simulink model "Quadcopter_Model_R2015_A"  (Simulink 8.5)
settings: Solver=ode45  SolverMode=SingleTasking  StartTime=0.0  StopTime=runtime  RelTol=1e-3
InitFcn:
  | clear mex
  | delete test_model_sfun.mexw64
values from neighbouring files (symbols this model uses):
  g = 9.81    [modelParameters.m]    (also in analyzeIMU_data.m = 9.8; getMomentOfInertia.m = 9.80665)
  height_controlled_o = dataStruct.RC_Throttle_Constant.data(1)    [modelParameters.m]
  If = 0.3836    [modelParameters.m]    (also in thrustDragConstantCalculations.m = [If0; If1; If2; If3]; Kd_error.m = I_0 * sign(rotor_speed_0) + I_1 * rotor_speed_0 + I_2 * roto)
  Jreq = 4.2012e-05    [modelParameters.m]
  Jxx = 0.0130    (= 0.013)    [modelParameters.m]
  Jyy = 0.0140    (= 0.014)    [modelParameters.m]
  Jzz = 0.0285    [modelParameters.m]
  Kd = 1.4852e-07    [modelParameters.m]    (also in calcDragConstant.m = ((A'*A)^-1)*A'*b; thrustDragConstantCalculations.m = calcDragConstant(data, Pmin, Pmax, Rm, Kv, Kq, If); Kd_error.m = 1.0317e-07)
  Kq = 96.3422    [modelParameters.m]    (also in thrustDragConstantCalculations.m; Kd_error.m)
  Kt = 1.2007e-05    [modelParameters.m]    (also in calcThrustConstant.m = ((A'*A)^(-1))*(A'*T); thrustDragConstantCalculations.m = calcThrustConstant(data))
  Kv = 96.3422    [modelParameters.m]    (also in thrustDragConstantCalculations.m; Kd_error.m)
  m = 1.140    (= 1.14)    [modelParameters.m]
  omega0_o = (sqrt(((height_controlled_o      - Pmin)/(Pmax - Pmin)* Vb - Rm * If) * 4 *      Rm * Kv^2 * Kq * Kd + 1) - 1) / (2 * Rm *       Kv * Kq * Kd)    [modelParameters.m]
  omega1_o = omega0_o    [modelParameters.m]
  omega2_o = omega0_o    [modelParameters.m]
  omega3_o = omega0_o    [modelParameters.m]
  pitch_o = pitch_measured_VRPN(1)    [modelParameters.m]
  pitchrate_o = (pitch_measured_VRPN(1) - pitch_measured_VRPN(2))/(time(1) - time(2))    [modelParameters.m]
  Pmax = 2e5    (= 200000)    [modelParameters.m]    (also in thrustDragConstantCalculations.m; Kd_error.m)
  Pmin = 1e5    (= 100000)    [modelParameters.m]    (also in thrustDragConstantCalculations.m; Kd_error.m)
  rhx = 0.16    [modelParameters.m]
  rhy = 0.16    [modelParameters.m]
  rhz = 0.03    [modelParameters.m]
  Rm = 0.2308    [modelParameters.m]    (also in thrustDragConstantCalculations.m; Kd_error.m)
  roll_o = roll_measured_VRPN(1)    [modelParameters.m]
  rollrate_o = (roll_measured_VRPN(1) - roll_measured_VRPN(2))/(time(1) - time(2))    [modelParameters.m]
  Tc = 0.04    [modelParameters.m]
  Tq = 0.005    [modelParameters.m]
  Vb = 11.4    [modelParameters.m]    (also in calcDragConstant.m = [data.(6); data.(6); data.(6); data.(6)]; Kd_error.m = data.(6))
  x_controlled_o = 0    [modelParameters.m]
  x_o = x_position(1)    [modelParameters.m]
  x_vel_o = (x_position(1) - x_position(2))/(time(1) - time(2))    [modelParameters.m]
  y_controlled_o = 0    [modelParameters.m]
  y_o = y_position(1)    [modelParameters.m]
  y_vel_o = (y_position(1) - y_position(2))/(time(1) - time(2))    [modelParameters.m]
  yaw_controlled_o = 0    [modelParameters.m]
  yaw_o = 0    [modelParameters.m]
  yawrate_o = 0    [modelParameters.m]
  z_o = z_position(1)    [modelParameters.m]
  z_vel_o = (z_position(1) - z_position(2))/(time(1) - time(2))    [modelParameters.m]
undefined symbols (not defined in the file or in its folder): DiscIntNeverNeededParam
libraries: simulink x12, vrlib x2
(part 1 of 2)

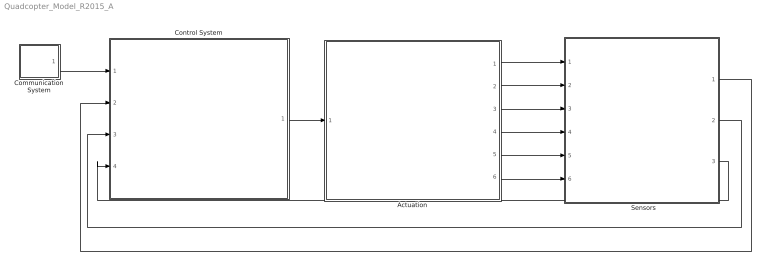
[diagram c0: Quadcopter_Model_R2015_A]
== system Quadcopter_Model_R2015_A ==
  "     Sensors   " : Subsystem
  Actuation : Subsystem
  Communication System : Subsystem
  Control System : Subsystem
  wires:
  Control System/1(P) -> Actuation/1(P)
  Communication System/1(setpoints) -> Control System/1(setpoints)
  Actuation/1(B_omega) -> "     Sensors   "/1(B_Omega)
  Actuation/2(euler_angles) -> "     Sensors   "/2(euler_angles)
  Actuation/3(B_vo) -> "     Sensors   "/3(B_vo)
  Actuation/4(E_ro) -> "     Sensors   "/4(E_ro)
  Actuation/5(B_vo_dot) -> "     Sensors   "/5(B_vo_dot)
  Actuation/6(B_g) -> "     Sensors   "/6(B_g)
  "     Sensors   "/3(current_position) -> Control System/4(current_position)
  "     Sensors   "/2(euler_rates) -> Control System/3(euler_rates)
  "     Sensors   "/1(euler_angles_filtered) -> Control System/2(euler_angles_filtered)

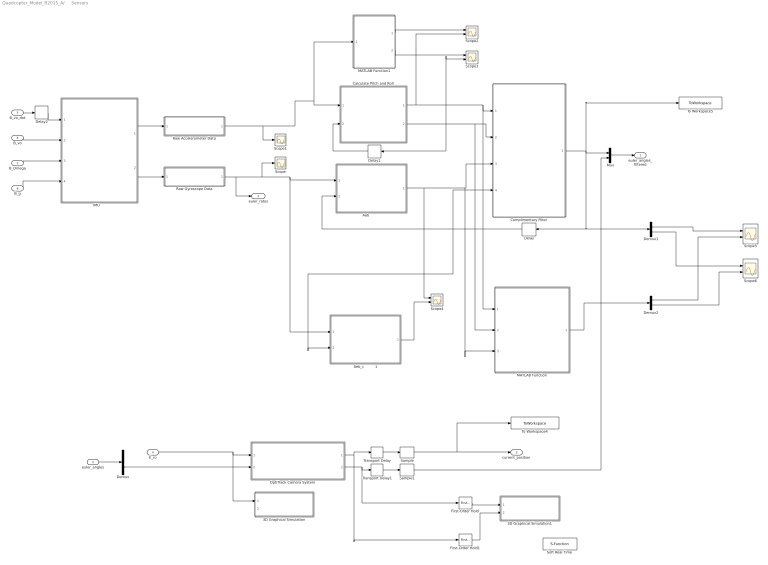
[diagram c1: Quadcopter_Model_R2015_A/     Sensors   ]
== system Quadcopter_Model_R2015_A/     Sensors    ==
  B_Omega : Inport
  euler_angles : Inport  Port=2
  B_vo : Inport  Port=3
  E_ro : Inport  Port=4
  B_vo_dot : Inport  Port=5
  B_g : Inport  Port=6
  3D Graphical Simulation : Subsystem  Commented=on
  3D Graphical Simulation1 : Subsystem  Commented=on
  "Aeb          " : MATLAB Function  TreatAsAtomicUnit=on
  Aeb_c          1 : MATLAB Function  TreatAsAtomicUnit=on
  Calculate Pitch and Roll : MATLAB Function  TreatAsAtomicUnit=on
  Complimentary Filter : MATLAB Function  TreatAsAtomicUnit=on
  Delay : Delay  DelayLength=1  InitialCondition=0
  Delay1 : Delay  DelayLength=1  InitialCondition=0  SampleTime=Tq
  Delay2 : Delay  DelayLength=1  InitialCondition=0  SampleTime=Tq
  Demux : Demux  Outputs=3
  Demux1 : Demux  Outputs=2
  Demux2 : Demux  Outputs=2
  First-Order Hold : simulink/Discrete/First-Order Hold  DisableCoverage=on  Ts=5e-3
  First-Order Hold1 : simulink/Discrete/First-Order Hold  DisableCoverage=on  Ts=5e-3
  "IMU      " : Subsystem
  MATLAB Function : MATLAB Function  TreatAsAtomicUnit=on
  MATLAB Function1 : MATLAB Function  TreatAsAtomicUnit=on
  Mux : Mux  Inputs=2
  "OptiTrack Camera System         " : Subsystem
  Raw Accelerometer Data : Subsystem  Variant=on
  Raw Gyroscope Data : Subsystem  Variant=on
  Sample : ZeroOrderHold  SampleTime=Tc
  Sample1 : ZeroOrderHold  SampleTime=Tc
  Scope : Scope
  Scope1 : Scope
  Scope{2..6} (5 alike) : Scope  NumInputPorts=2
  Soft Real Time : S-Function  Commented=on  FunctionName=sfun_time  Parameters=x  SFunctionDeploymentMode=off  EnableBusSupport=off
  To Workspace4 : ToWorkspace  VariableName=position_model  SaveFormat=Structure With Time  SampleTime=Tc
  To Workspace5 : ToWorkspace  VariableName=angle_IMU_reading  SaveFormat=Structure With Time  SampleTime=Tq
  Transport Delay : TransportDelay  DelayTime=6e-3
  Transport Delay1 : TransportDelay  DelayTime=6e-3
  euler_angles_filtered : Outport
  euler_rates : Outport  Port=2
  current_position : Outport  Port=3
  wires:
  "IMU      "/1(accelerometer) -> Raw Accelerometer Data/1(raw_accel_model)
  "IMU      "/2(gyroscope) -> Raw Gyroscope Data/1(raw_gyro_model)
  B_vo/1 -> "IMU      "/2(B_vo)
  B_Omega/1 -> "IMU      "/3(B_Omega)
  B_g/1 -> "IMU      "/4(B_g)
  Calculate Pitch and Roll/2(accel_roll) -> Scope3/2, Delay1/1, MATLAB Function/2(accel_roll), Complimentary Filter/2(accel_roll)
  Calculate Pitch and Roll/1(accel_pitch) -> Scope2/2, MATLAB Function/1(accel_pitch), Complimentary Filter/1(accel_pitch)
  Delay1/1 -> Calculate Pitch and Roll/2(accel_roll_prev)
  First-Order Hold/1 -> 3D Graphical Simulation1/1("Euler Angles ")
  E_ro/1 -> 3D Graphical Simulation/1(Displacement), "OptiTrack Camera System         "/1(E_ro)
  First-Order Hold1/1 -> 3D Graphical Simulation1/2(Displacement)
  B_vo_dot/1 -> Delay2/1
  Delay2/1 -> "IMU      "/1(B_vo_dot)
  "OptiTrack Camera System         "/1(E_ro_camera) -> Transport Delay/1, First-Order Hold1/1
  "OptiTrack Camera System         "/2(yaw_camera) -> First-Order Hold/1, Transport Delay1/1
  Transport Delay/1 -> Sample/1
  Transport Delay1/1 -> Sample1/1
  Sample/1 -> To Workspace4/1, current_position/1
  Raw Accelerometer Data/1(raw_accel) -> MATLAB Function1/1(accel_reading), Calculate Pitch and Roll/1(accel_reading), Scope1/1
  Raw Gyroscope Data/1(raw_gyro) -> Aeb_c          1/1(gyro_reading), "Aeb          "/1(gyro_reading), Scope/1, euler_rates/1
  Delay/1 -> Complimentary Filter/4(prev_euler_angles), Aeb_c          1/2(euler_angles_filtered), "Aeb          "/2(euler_angles_filtered)
  euler_angles/1 -> Demux/1
  Demux/3 -> "OptiTrack Camera System         "/2(yaw)
  Sample1/1 -> Mux/2
  Mux/1 -> euler_angles_filtered/1
  Complimentary Filter/1(euler_angles_IMU) -> Mux/1, To Workspace5/1, Demux1/1, Delay/1
  "Aeb          "/1(euler_rates_IMU) -> Scope4/1, MATLAB Function/3(euler_rates_gyro), Complimentary Filter/3(euler_rates_gyro)
  Aeb_c          1/1(euler_rates_IMU) -> Scope4/2
  MATLAB Function/1(euler_angles_IMU) -> Demux2/1
  Demux1/1 -> Scope5/1
  Demux2/1 -> Scope5/2
  Demux1/2 -> Scope6/1
  Demux2/2 -> Scope6/2
  MATLAB Function1/1(accel_pitch) -> Scope2/1
  MATLAB Function1/2(accel_roll) -> Scope3/1

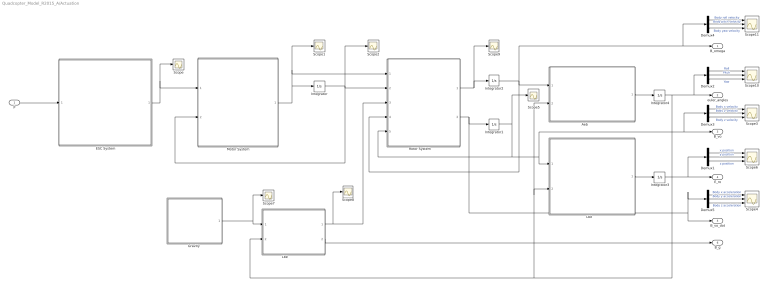
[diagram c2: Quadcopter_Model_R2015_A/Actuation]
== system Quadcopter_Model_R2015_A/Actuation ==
  P : Inport
  "Aeb               " : MATLAB Function  TreatAsAtomicUnit=on
  Demux{1..5} (5 alike) : Demux  Outputs=3
  ESC System : MATLAB Function  TreatAsAtomicUnit=on
  "Gravity  " : MATLAB Function  TreatAsAtomicUnit=on
  Integrator : Integrator  InitialCondition=[omega0_o, omega1_o, omega2_o, omega3_o]
  Integrator1 : Integrator  InitialCondition=[x_vel_o; y_vel_o; z_vel_o]
  Integrator2 : Integrator  InitialCondition=[rollrate_o; pitchrate_o; yawrate_o]
  Integrator3 : Integrator  InitialCondition=[x_o; y_o; z_o]
  Integrator4 : Integrator  InitialCondition=[roll_o; pitch_o; yaw_o]  ContinuousStateAttributes=['phi' 'theta' 'psi']
  "Lbe      " : MATLAB Function  TreatAsAtomicUnit=on
  "Lbe                  " : MATLAB Function  TreatAsAtomicUnit=on
  Motor System : MATLAB Function  TreatAsAtomicUnit=on
  "Rotor System        " : MATLAB Function  TreatAsAtomicUnit=on
  Scope{,1..2,5,7..9} (7 alike) : Scope
  Scope{3..4,6,10..11} (5 alike) : Scope  NumInputPorts=3
  B_omega : Outport
  euler_angles : Outport  Port=2
  B_vo : Outport  Port=3
  E_ro : Outport  Port=4
  B_vo_dot : Outport  Port=5
  B_g : Outport  Port=6
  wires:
  ESC System/1(Vb_eff) -> Scope/1, Motor System/1(Vb_eff)
  Motor System/1(w_dot) -> Integrator/1, "Rotor System        "/1(w_dot), Scope1/1
  "Rotor System        "/1(B_omega_dot) -> Scope9/1, Integrator2/1
  Integrator2/1 -> "Rotor System        "/4(B_omega), B_omega/1, Demux4/1, "Aeb               "/1(B_omega)
  "Aeb               "/1(euler_rates) -> Integrator4/1
  "Lbe      "/1(E_ro) -> Integrator3/1
  Integrator3/1 -> Demux1/1, E_ro/1
  "Lbe                  "/1(B_Fg) -> Scope8/1, "Rotor System        "/3(B_Fg)
  "Lbe                  "/2(B_g) -> B_g/1
  Demux1/2 -> Scope6/2  "y position"
  Demux1/1 -> Scope6/1  "x position"
  Demux1/3 -> Scope6/3  "z position"
  Demux2/2 -> Scope10/2  "Pitch"
  Demux2/1 -> Scope10/1  "Roll"
  Demux2/3 -> Scope10/3  "Yaw"
  Demux4/2 -> Scope11/2  "Body pitch velocity"
  Demux4/1 -> Scope11/1  "Body roll velocity"
  Demux4/3 -> Scope11/3  "Body yaw velocity"
  Demux3/2 -> Scope3/2  "Body y velocity"
  Demux3/1 -> Scope3/1  "Body x velocity"
  Demux3/3 -> Scope3/3  "Body z velocity"
  Demux5/2 -> Scope4/2  "Body y acceleration"
  Demux5/1 -> Scope4/1  "Body x acceleration"
  Demux5/3 -> Scope4/3  "Body z acceleration"
  Integrator1/1 -> Scope5/1, "Rotor System        "/5(B_vo), "Lbe      "/1(B_vo), Demux3/1, B_vo/1
  "Rotor System        "/2(B_vo_dot) -> Demux5/1, B_vo_dot/1, Integrator1/1
  Integrator4/1 -> euler_angles/1, Demux2/1, "Lbe      "/2(euler_angles), "Aeb               "/2(euler_angles), "Lbe                  "/2(euler_angles)
  P/1 -> ESC System/1(P)
  "Gravity  "/1(E_Fg) -> Scope7/1, "Lbe                  "/1(E_Fg)
  Integrator/1 -> Motor System/2(w), "Rotor System        "/2(w), Scope2/1

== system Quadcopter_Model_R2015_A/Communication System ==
  Step : Step  Before=[0; 0; 0; 0]  After=[0; 0; 0; 0]  SampleTime=Tq
  setpoints : Outport
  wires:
  Step/1 -> setpoints/1

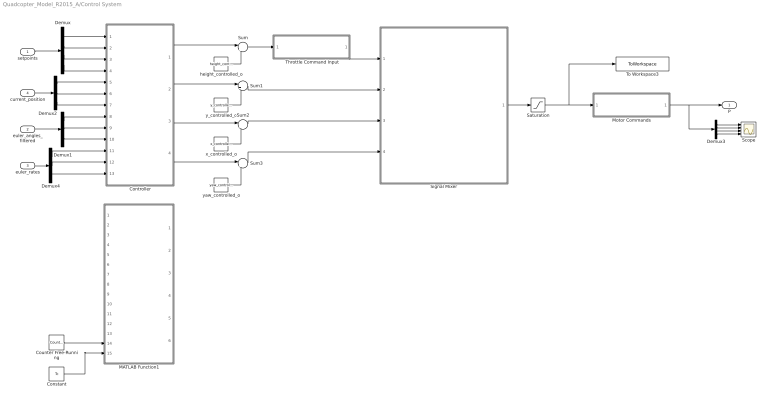
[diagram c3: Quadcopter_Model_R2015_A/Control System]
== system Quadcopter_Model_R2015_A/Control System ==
  setpoints : Inport
  euler_angles_filtered : Inport  Port=2
  euler_rates : Inport  Port=3
  current_position : Inport  Port=4
  Constant : Constant  Value=Tc  SampleTime=Tc
  Controller : Subsystem
  Counter Free-Running : simulink/Sources/Counter Free-Running  NumBits=32  tsamp=Tc
  Demux : Demux
  Demux1 : Demux  Outputs=3
  Demux2 : Demux  Outputs=3
  Demux3 : Demux
  Demux4 : Demux  Outputs=3
  MATLAB Function1 : MATLAB Function  Commented=on  TreatAsAtomicUnit=on  SystemSampleTime=Tq
  Motor Commands : Subsystem  Variant=on
  Saturation : Saturate  UpperLimit=Pmax*ones(4,1)  LowerLimit=Pmin*ones(4,1)
  Scope : Scope  NumInputPorts=4
  Signal Mixer : MATLAB Function  TreatAsAtomicUnit=on
  Sum{,1..3} (4 alike) : Sum  Inputs=|++
  Throttle Command Input : Subsystem  Variant=on
  To Workspace3 : ToWorkspace  VariableName=motorCommands  SaveFormat=Structure With Time  SampleTime=Tq
  height_controlled_o : Constant  Value=height_controlled_o  SampleTime=Tc
  x_controlled_o : Constant  Value=x_controlled_o
  y_controlled_o : Constant  Value=y_controlled_o
  yaw_controlled_o : Constant  Value=yaw_controlled_o
  P : Outport
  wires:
  setpoints/1 -> Demux/1
  euler_angles_filtered/1 -> Demux1/1
  current_position/1 -> Demux2/1
  euler_rates/1 -> Demux4/1
  Demux/1 -> Controller/1(x_setpoint)
  Demux/2 -> Controller/2(y_setpoint)
  Demux/3 -> Controller/3(z_setpoint)
  Demux2/1 -> Controller/5(x_position)
  Demux2/2 -> Controller/6(y_position)
  Demux2/3 -> Controller/7(z_position)
  Controller/2(y_controlled) -> Sum1/1
  Controller/4(yaw_controlled) -> Sum3/1
  y_controlled_o/1 -> Sum1/2
  x_controlled_o/1 -> Sum2/2
  yaw_controlled_o/1 -> Sum3/2
  Signal Mixer/1(P) -> Saturation/1
  Demux1/1 -> Controller/8(roll)
  Demux1/2 -> Controller/9(pitch)
  Demux4/1 -> Controller/11(roll_rate)
  Demux4/2 -> Controller/12(pitch_rate)
  Demux4/3 -> Controller/13(yaw_rate)
  Demux/4 -> Controller/4(yaw_setpoint)
  Demux1/3 -> Controller/10(yaw)
  Controller/3(x_controlled) -> Sum2/1
  Counter Free-Running/1 -> MATLAB Function1/14(vrpn_id)
  Constant/1 -> MATLAB Function1/15(Tc)
  Sum1/1 -> Signal Mixer/2(y_controlled)
  Sum2/1 -> Signal Mixer/3(x_controlled)
  Sum3/1 -> Signal Mixer/4(yaw_controlled)
  Throttle Command Input/1(z_command) -> Signal Mixer/1(height_controlled)
  Controller/1(height_controlled) -> Sum/1
  height_controlled_o/1 -> Sum/2
  Motor Commands/1(z_command) -> Demux3/1, P/1
  Demux3/1 -> Scope/1
  Demux3/2 -> Scope/2
  Demux3/3 -> Scope/3
  Demux3/4 -> Scope/4
  Sum/1 -> Throttle Command Input/1(z_command_model)
  Saturation/1 -> To Workspace3/1, Motor Commands/1(z_command_model)

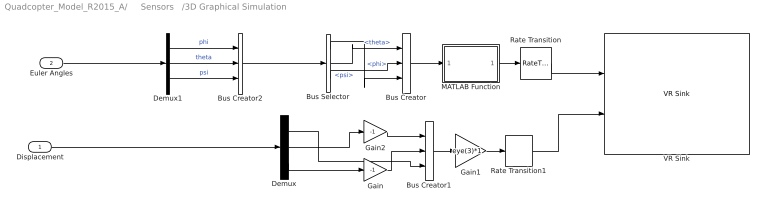
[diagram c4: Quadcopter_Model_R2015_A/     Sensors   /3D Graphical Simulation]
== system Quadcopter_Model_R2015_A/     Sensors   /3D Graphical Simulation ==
  Displacement : Inport
  Euler Angles : Inport  Port=2
  Bus Creator : BusCreator  Inputs=3
  Bus Creator1 : BusCreator  Inputs=3
  Bus Creator2 : BusCreator  Inputs=3
  Bus Selector : BusSelector  OutputSignals=phi,theta,psi
  Demux : Demux  Outputs=3
  Demux1 : Demux  Outputs=3
  Gain : Gain  Gain=-1
  Gain1 : Gain  Gain=eye(3)*1  Multiplication=Matrix(K*u)
  Gain2 : Gain  Gain=-1
  MATLAB Function : MATLAB Function  TreatAsAtomicUnit=on
  Rate Transition : RateTransition  OutPortSampleTime=0.06
  Rate Transition1 : RateTransition  OutPortSampleTime=0.06
  VR Sink : vrlib/VR Sink  InstantiateOnLoad=on  SampleTime=-1  ViewEnable=on  RemoteChange=off  RemoteView=off  FieldsWritten=Helicopter.rotation.4.1.1.double#Helicopter.translation.3.1.1.double  WorldFileName=quadrotor_world_ucart.wrl  AutoView=on  VideoDimensions=[]  AllowVariableSize=off
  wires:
  Displacement/1 -> Demux/1
  Bus Creator2/1 -> Bus Selector/1
  Demux/1 -> Bus Creator1/3
  Gain/1 -> Bus Creator1/2
  Gain2/1 -> Bus Creator1/1
  Rate Transition1/1 -> VR Sink/2
  Rate Transition/1 -> VR Sink/1
  Demux/3 -> Gain/1
  Demux/2 -> Gain2/1
  Bus Creator1/1 -> Gain1/1
  Bus Selector/1 -> Bus Creator/3  "<phi>"
  Bus Selector/3 -> Bus Creator/2  "<psi>"
  Bus Selector/2 -> Bus Creator/1  "<theta>"
  Gain1/1 -> Rate Transition1/1
  Demux1/3 -> Bus Creator2/3  "psi"
  Demux1/2 -> Bus Creator2/2  "theta"
  Demux1/1 -> Bus Creator2/1  "phi"
  Euler Angles/1 -> Demux1/1
  Bus Creator/1 -> MATLAB Function/1(u)
  MATLAB Function/1(y) -> Rate Transition/1

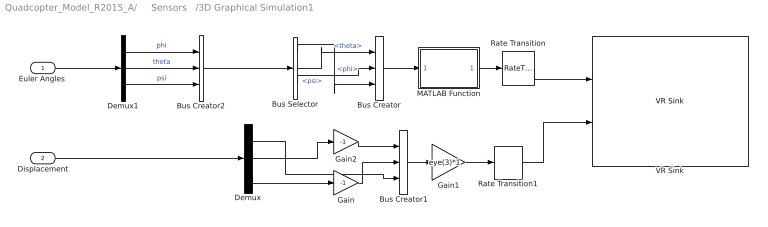
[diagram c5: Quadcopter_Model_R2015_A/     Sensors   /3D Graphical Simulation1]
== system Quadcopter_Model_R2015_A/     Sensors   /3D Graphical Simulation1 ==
  "Euler Angles " : Inport
  Displacement : Inport  Port=2
  Bus Creator : BusCreator  Inputs=3
  Bus Creator1 : BusCreator  Inputs=3
  Bus Creator2 : BusCreator  Inputs=3
  Bus Selector : BusSelector  OutputSignals=phi,theta,psi
  Demux : Demux  Outputs=3
  Demux1 : Demux  Outputs=3
  Gain : Gain  Gain=-1
  Gain1 : Gain  Gain=eye(3)*1  Multiplication=Matrix(K*u)
  Gain2 : Gain  Gain=-1
  MATLAB Function : MATLAB Function  TreatAsAtomicUnit=on
  Rate Transition : RateTransition  OutPortSampleTime=0.06
  Rate Transition1 : RateTransition  OutPortSampleTime=0.06
  VR Sink : vrlib/VR Sink  InstantiateOnLoad=on  SampleTime=-1  ViewEnable=on  RemoteChange=off  RemoteView=off  FieldsWritten=Helicopter.rotation.4.1.1.double#Helicopter.translation.3.1.1.double  WorldFileName=quadrotor_world_ucart.wrl  AutoView=on  VideoDimensions=[]  AllowVariableSize=off
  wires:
  Bus Creator2/1 -> Bus Selector/1
  Demux/1 -> Bus Creator1/3
  Gain/1 -> Bus Creator1/2
  Gain2/1 -> Bus Creator1/1
  Rate Transition1/1 -> VR Sink/2
  Rate Transition/1 -> VR Sink/1
  Demux/3 -> Gain/1
  Demux/2 -> Gain2/1
  Bus Creator1/1 -> Gain1/1
  Bus Selector/1 -> Bus Creator/3  "<phi>"
  Bus Selector/3 -> Bus Creator/2  "<psi>"
  Bus Selector/2 -> Bus Creator/1  "<theta>"
  Gain1/1 -> Rate Transition1/1
  Demux1/3 -> Bus Creator2/3  "psi"
  Demux1/2 -> Bus Creator2/2  "theta"
  Demux1/1 -> Bus Creator2/1  "phi"
  Bus Creator/1 -> MATLAB Function/1(u)
  MATLAB Function/1(y) -> Rate Transition/1
  Displacement/1 -> Demux/1
  "Euler Angles "/1 -> Demux1/1

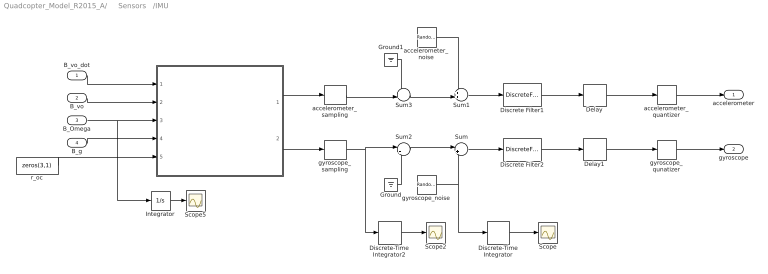
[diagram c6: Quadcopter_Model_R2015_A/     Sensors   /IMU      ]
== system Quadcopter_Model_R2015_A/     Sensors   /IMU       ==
  B_vo_dot : Inport
  B_vo : Inport  Port=2
  B_Omega : Inport  Port=3
  B_g : Inport  Port=4
  "       " : MATLAB Function  TreatAsAtomicUnit=on
  Delay : Delay  Commented=through  DelayLength=4  InitialCondition=0  SampleTime=Tq
  Delay1 : Delay  Commented=through  DelayLength=4  InitialCondition=0  SampleTime=Tq
  Discrete Filter1 : DiscreteFilter  Numerator=[0 0.1454]  Denominator=[1 -0.8546]  InitialStates=[0, 0, -1]  SampleTime=Tq
  Discrete Filter2 : DiscreteFilter  Numerator=[0 0.1454]  Denominator=[1 -0.8546]  SampleTime=Tq
  Discrete-Time Integrator : DiscreteIntegrator  InitialConditionSetting=State (most efficient)  SampleTime=-1  ICPrevOutput=DiscIntNeverNeededParam  ICPrevScaledInput=DiscIntNeverNeededParam
  Discrete-Time Integrator2 : DiscreteIntegrator  InitialConditionSetting=State (most efficient)  SampleTime=-1  ICPrevOutput=DiscIntNeverNeededParam  ICPrevScaledInput=DiscIntNeverNeededParam
  Ground : Ground
  Ground1 : Ground
  Integrator : Integrator
  Scope : Scope
  Scope2 : Scope
  Scope5 : Scope
  Sum : Sum  Inputs=|++
  Sum1 : Sum  Inputs=++|
  Sum2 : Sum  Inputs=|++
  Sum3 : Sum  Inputs=++|
  accelerometer_noise : RandomNumber  Mean=zeros(3,1)  Variance=[ 3e-7 ; 3.3e-7 ; 7.2e-7 ]  Seed=[0,1,2]  SampleTime=Tq
  accelerometer_quantizer : Quantizer  QuantizationInterval=2.4400e-04
  accelerometer_sampling : ZeroOrderHold  SampleTime=Tq
  gyroscope_noise : RandomNumber  Mean=zeros(3,1)  Variance=[ 2.2e-8 ; 1.1e-7 ; 2.4e-8 ]  Seed=[0,1,2]  SampleTime=Tq
  gyroscope_qunatizer : Quantizer  QuantizationInterval=1.1e-3
  gyroscope_sampling : ZeroOrderHold  SampleTime=Tq
  r_oc : Constant  Value=zeros(3,1)
  accelerometer : Outport
  gyroscope : Outport  Port=2
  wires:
  accelerometer_noise/1 -> Sum1/1
  Sum2/1 -> Sum/1
  Sum3/1 -> Sum1/2
  gyroscope_noise/1 -> Sum/2, Discrete-Time Integrator/1
  gyroscope_sampling/1 -> Sum2/1, Discrete-Time Integrator2/1
  accelerometer_sampling/1 -> Sum3/2
  Ground/1 -> Sum2/2
  Ground1/1 -> Sum3/1
  B_vo_dot/1 -> "       "/1(B_vo_dot)
  B_vo/1 -> "       "/2(B_vo)
  B_Omega/1 -> Integrator/1, "       "/3(B_Omega)
  B_g/1 -> "       "/4(B_g)
  r_oc/1 -> "       "/5(r_oc)
  "       "/2(gyroReading) -> gyroscope_sampling/1
  "       "/1(accelReading) -> accelerometer_sampling/1
  Discrete-Time Integrator/1 -> Scope/1
  Discrete-Time Integrator2/1 -> Scope2/1
  Integrator/1 -> Scope5/1
  Sum1/1 -> Discrete Filter1/1
  Sum/1 -> Discrete Filter2/1
  accelerometer_quantizer/1 -> accelerometer/1
  gyroscope_qunatizer/1 -> gyroscope/1
  Discrete Filter1/1 -> Delay/1
  Discrete Filter2/1 -> Delay1/1
  Delay/1 -> accelerometer_quantizer/1
  Delay1/1 -> gyroscope_qunatizer/1

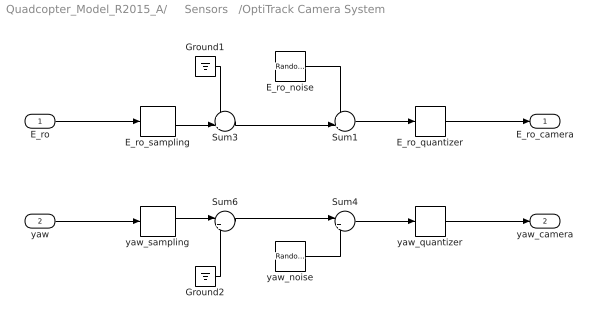
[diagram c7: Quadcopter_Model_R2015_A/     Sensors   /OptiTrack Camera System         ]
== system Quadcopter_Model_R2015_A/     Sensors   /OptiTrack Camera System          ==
  E_ro : Inport
  yaw : Inport  Port=2
  E_ro_noise : RandomNumber  Mean=zeros(3,1)  Variance=[ 7.9664e-10 ; 1.1928e-10 ; 5.0636e-10 ]  Seed=[0,1,2]  SampleTime=Tc
  E_ro_quantizer : Quantizer  QuantizationInterval=2.4400e-04
  E_ro_sampling : ZeroOrderHold  SampleTime=Tc
  Ground1 : Ground
  Ground2 : Ground
  Sum1 : Sum  Inputs=++|
  Sum3 : Sum  Inputs=++|
  Sum4 : Sum  Inputs=|++
  Sum6 : Sum  Inputs=|++
  yaw_noise : RandomNumber  Variance=1.0783e-9  SampleTime=Tc
  yaw_quantizer : Quantizer  QuantizationInterval=1.1e-3
  yaw_sampling : ZeroOrderHold  SampleTime=Tc
  E_ro_camera : Outport
  yaw_camera : Outport  Port=2
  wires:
  E_ro_noise/1 -> Sum1/1
  Sum3/1 -> Sum1/2
  Sum1/1 -> E_ro_quantizer/1
  E_ro_sampling/1 -> Sum3/2
  Ground1/1 -> Sum3/1
  Sum4/1 -> yaw_quantizer/1
  Sum6/1 -> Sum4/1
  yaw_noise/1 -> Sum4/2
  yaw_sampling/1 -> Sum6/1
  Ground2/1 -> Sum6/2
  yaw/1 -> yaw_sampling/1
  E_ro/1 -> E_ro_sampling/1
  E_ro_quantizer/1 -> E_ro_camera/1
  yaw_quantizer/1 -> yaw_camera/1

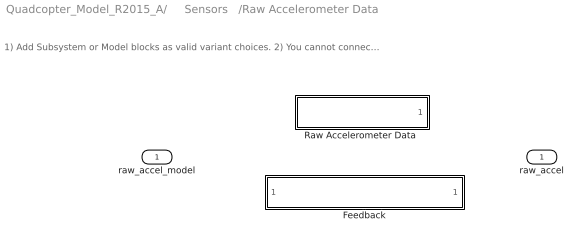
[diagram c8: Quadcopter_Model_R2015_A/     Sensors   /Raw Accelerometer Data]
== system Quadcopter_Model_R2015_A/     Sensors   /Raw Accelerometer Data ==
  note: 1) Add Subsystem or Model blocks as valid variant choices. 2) You cannot connect blocks at this level. At simulation, connectivity is automatically determined, based on the active variant and port name matching.
  raw_accel_model : Inport
  Feedback : Subsystem  VariantControl=logAnalysisToggle==0
  "Raw Accelerometer Data " : Subsystem  VariantControl=logAnalysisToggle==1
  raw_accel : Outport

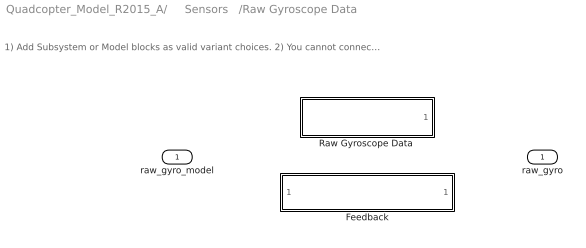
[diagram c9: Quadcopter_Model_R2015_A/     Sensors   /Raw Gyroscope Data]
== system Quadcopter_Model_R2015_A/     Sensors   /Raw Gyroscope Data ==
  note: 1) Add Subsystem or Model blocks as valid variant choices. 2) You cannot connect blocks at this level. At simulation, connectivity is automatically determined, based on the active variant and port name matching.
  raw_gyro_model : Inport
  Feedback : Subsystem  VariantControl=logAnalysisToggle==0
  "Raw Gyroscope Data " : Subsystem  VariantControl=logAnalysisToggle==1
  raw_gyro : Outport

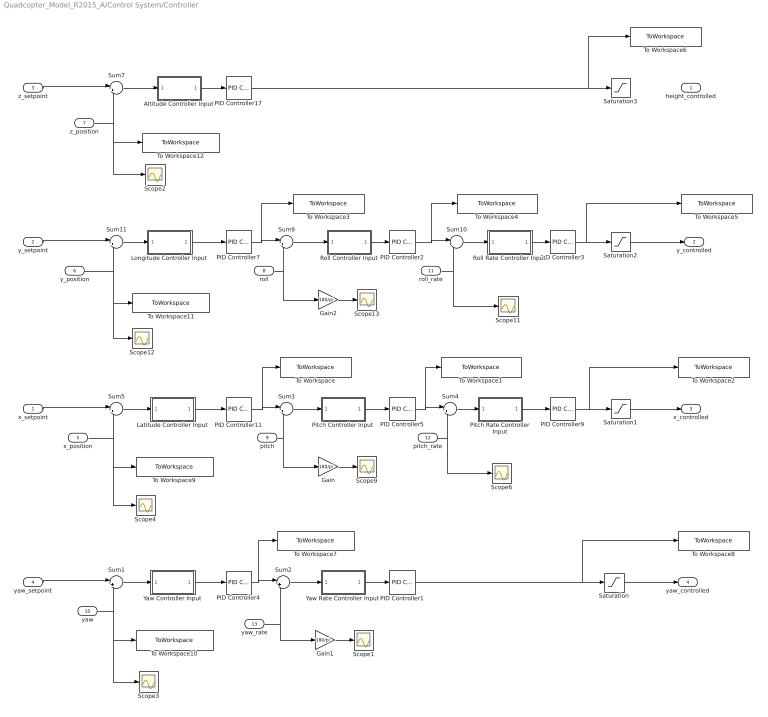
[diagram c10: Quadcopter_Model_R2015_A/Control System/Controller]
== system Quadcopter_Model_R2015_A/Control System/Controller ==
  x_setpoint : Inport
  y_setpoint : Inport  Port=2
  z_setpoint : Inport  Port=3
  yaw_setpoint : Inport  Port=4
  x_position : Inport  Port=5
  y_position : Inport  Port=6
  z_position : Inport  Port=7
  roll : Inport  Port=8
  pitch : Inport  Port=9
  yaw : Inport  Port=10
  roll_rate : Inport  Port=11
  pitch_rate : Inport  Port=12
  yaw_rate : Inport  Port=13
  Altitude Controller Input : Subsystem  Variant=on
  Gain : Gain  Gain=180/pi
  Gain1 : Gain  Gain=180/pi
  Gain2 : Gain  Gain=180/pi
  Latitude Controller Input : Subsystem  Variant=on
  Longitude Controller Input : Subsystem  Variant=on
  PID Controller1 : simulink/Continuous/PID Controller  Controller=P  TimeDomain=Discrete-time  SampleTime=Tq  IntegratorMethod=Forward Euler  FilterMethod=Forward Euler  Form=Parallel  UseFilter=on  ControllerParametersSource=internal  P=29700  I=-77.7  D=2.32  N=1/0.0818  InitialConditionSource=internal  InitialConditionForIntegrator=0  InitialConditionForFilter=0  ExternalReset=none  ZeroCross=off  LimitOutput=off  UpperSaturationLimit=inf  LowerSaturationLimit=-inf  LinearizeAsGain=on  AntiWindupMode=none  Kb=1  TrackingMode=off  Kt=1  PParamMin=[]  PParamMax=[]  IParamMin=[]  IParamMax=[]  DParamMin=[]  DParamMax=[]  NParamMin=[]  NParamMax=[]  KbParamMin=[]  KbParamMax=[]  KtParamMin=[]  KtParamMax=[]  POutMin=[]  POutMax=[]  IOutMin=[]  IOutMax=[]  DOutMin=[]  DOutMax=[]  NOutMin=[]  NOutMax=[]  KbOutMin=[]  KbOutMax=[]  KtOutMin=[]  KtOutMax=[]  IntegratorOutMin=[]  IntegratorOutMax=[]  FilterOutMin=[]  FilterOutMax=[]  SumOutMin=[]  SumOutMax=[]  SumI1OutMin=[]  SumI1OutMax=[]  SumI2OutMin=[]  SumI2OutMax=[]  SumI3OutMin=[]  SumI3OutMax=[]  SumDOutMin=[]  SumDOutMax=[]  SaturationOutMin=[]  SaturationOutMax=[]  IntegratorContinuousStateAttributes=''  IntegratorStateMustResolveToSignalObject=off  IntegratorRTWStateStorageClass=Auto  FilterContinuousStateAttributes=''  FilterStateMustResolveToSignalObject=off  FilterRTWStateStorageClass=Auto  DifferentiatorICPrevScaledInput=0  DifferentiatorOutMin=[]  DifferentiatorOutMax=[]
  PID Controller11 : simulink/Continuous/PID Controller  Controller=PID  TimeDomain=Discrete-time  SampleTime=Tc  IntegratorMethod=Forward Euler  FilterMethod=Forward Euler  Form=Parallel  UseFilter=on  ControllerParametersSource=internal  P=-0.015  I=0  D=-0.25  N=3  InitialConditionSource=internal  InitialConditionForIntegrator=0  InitialConditionForFilter=0  ExternalReset=none  LimitOutput=off  UpperSaturationLimit=inf  LowerSaturationLimit=-inf  LinearizeAsGain=on  AntiWindupMode=none  Kb=1  TrackingMode=off  Kt=1  PParamMin=[]  PParamMax=[]  IParamMin=[]  IParamMax=[]  DParamMin=[]  DParamMax=[]  NParamMin=[]  NParamMax=[]  KbParamMin=[]  KbParamMax=[]  KtParamMin=[]  KtParamMax=[]  POutMin=[]  POutMax=[]  IOutMin=[]  IOutMax=[]  DOutMin=[]  DOutMax=[]  NOutMin=[]  NOutMax=[]  KbOutMin=[]  KbOutMax=[]  KtOutMin=[]  KtOutMax=[]  IntegratorOutMin=[]  IntegratorOutMax=[]  FilterOutMin=[]  FilterOutMax=[]  SumOutMin=[]  SumOutMax=[]  SumI1OutMin=[]  SumI1OutMax=[]  SumI2OutMin=[]  SumI2OutMax=[]  SumI3OutMin=[]  SumI3OutMax=[]  SumDOutMin=[]  SumDOutMax=[]  SaturationOutMin=[]  SaturationOutMax=[]  IntegratorContinuousStateAttributes=''  IntegratorStateMustResolveToSignalObject=off  IntegratorRTWStateStorageClass=Auto  FilterContinuousStateAttributes=''  FilterStateMustResolveToSignalObject=off  FilterRTWStateStorageClass=Auto  DifferentiatorICPrevScaledInput=0  DifferentiatorOutMin=[]  DifferentiatorOutMax=[]
  PID Controller17 : simulink/Continuous/PID Controller  Controller=PID  TimeDomain=Discrete-time  SampleTime=Tc  IntegratorMethod=Forward Euler  FilterMethod=Forward Euler  Form=Parallel  UseFilter=off  ControllerParametersSource=internal  P=9804  I=817  D=7353  N=5.79502261645411  InitialConditionSource=internal  InitialConditionForIntegrator=0  InitialConditionForFilter=0  ExternalReset=none  LimitOutput=off  UpperSaturationLimit=inf  LowerSaturationLimit=-inf  LinearizeAsGain=on  AntiWindupMode=none  Kb=1  TrackingMode=off  Kt=1  PParamMin=[]  PParamMax=[]  IParamMin=[]  IParamMax=[]  DParamMin=[]  DParamMax=[]  NParamMin=[]  NParamMax=[]  KbParamMin=[]  KbParamMax=[]  KtParamMin=[]  KtParamMax=[]  POutMin=[]  POutMax=[]  IOutMin=[]  IOutMax=[]  DOutMin=[]  DOutMax=[]  NOutMin=[]  NOutMax=[]  KbOutMin=[]  KbOutMax=[]  KtOutMin=[]  KtOutMax=[]  IntegratorOutMin=[]  IntegratorOutMax=[]  FilterOutMin=[]  FilterOutMax=[]  SumOutMin=[]  SumOutMax=[]  SumI1OutMin=[]  SumI1OutMax=[]  SumI2OutMin=[]  SumI2OutMax=[]  SumI3OutMin=[]  SumI3OutMax=[]  SumDOutMin=[]  SumDOutMax=[]  SaturationOutMin=[]  SaturationOutMax=[]  IntegratorContinuousStateAttributes=''  IntegratorStateMustResolveToSignalObject=off  IntegratorRTWStateStorageClass=Auto  FilterContinuousStateAttributes=''  FilterStateMustResolveToSignalObject=off  FilterRTWStateStorageClass=Auto  DifferentiatorICPrevScaledInput=0  DifferentiatorOutMin=[]  DifferentiatorOutMax=[]
  PID Controller2 : simulink/Continuous/PID Controller  Controller=PD  TimeDomain=Discrete-time  SampleTime=Tq  IntegratorMethod=Forward Euler  FilterMethod=Forward Euler  Form=Parallel  UseFilter=off  ControllerParametersSource=internal  P=15  I=35.1207902652377  D=0.2  N=40.0107970227961  InitialConditionSource=internal  InitialConditionForIntegrator=0  InitialConditionForFilter=0  ExternalReset=none  LimitOutput=off  UpperSaturationLimit=inf  LowerSaturationLimit=-inf  LinearizeAsGain=on  AntiWindupMode=none  Kb=1  TrackingMode=off  Kt=1  PParamMin=[]  PParamMax=[]  IParamMin=[]  IParamMax=[]  DParamMin=[]  DParamMax=[]  NParamMin=[]  NParamMax=[]  KbParamMin=[]  KbParamMax=[]  KtParamMin=[]  KtParamMax=[]  POutMin=[]  POutMax=[]  IOutMin=[]  IOutMax=[]  DOutMin=[]  DOutMax=[]  NOutMin=[]  NOutMax=[]  KbOutMin=[]  KbOutMax=[]  KtOutMin=[]  KtOutMax=[]  IntegratorOutMin=[]  IntegratorOutMax=[]  FilterOutMin=[]  FilterOutMax=[]  SumOutMin=[]  SumOutMax=[]  SumI1OutMin=[]  SumI1OutMax=[]  SumI2OutMin=[]  SumI2OutMax=[]  SumI3OutMin=[]  SumI3OutMax=[]  SumDOutMin=[]  SumDOutMax=[]  SaturationOutMin=[]  SaturationOutMax=[]  IntegratorContinuousStateAttributes=''  IntegratorStateMustResolveToSignalObject=off  IntegratorRTWStateStorageClass=Auto  FilterContinuousStateAttributes=''  FilterStateMustResolveToSignalObject=off  FilterRTWStateStorageClass=Auto  DifferentiatorICPrevScaledInput=0  DifferentiatorOutMin=[]  DifferentiatorOutMax=[]
  PID Controller3 : simulink/Continuous/PID Controller  Controller=PD  TimeDomain=Discrete-time  SampleTime=Tq  IntegratorMethod=Forward Euler  FilterMethod=Forward Euler  Form=Parallel  UseFilter=off  ControllerParametersSource=internal  P=4600  I=1575.82088970639  D=550  N=244.660686071579  InitialConditionSource=internal  InitialConditionForIntegrator=0  InitialConditionForFilter=0  ExternalReset=none  LimitOutput=off  UpperSaturationLimit=inf  LowerSaturationLimit=-inf  LinearizeAsGain=on  AntiWindupMode=none  Kb=1  TrackingMode=off  Kt=1  PParamMin=[]  PParamMax=[]  IParamMin=[]  IParamMax=[]  DParamMin=[]  DParamMax=[]  NParamMin=[]  NParamMax=[]  KbParamMin=[]  KbParamMax=[]  KtParamMin=[]  KtParamMax=[]  POutMin=[]  POutMax=[]  IOutMin=[]  IOutMax=[]  DOutMin=[]  DOutMax=[]  NOutMin=[]  NOutMax=[]  KbOutMin=[]  KbOutMax=[]  KtOutMin=[]  KtOutMax=[]  IntegratorOutMin=[]  IntegratorOutMax=[]  FilterOutMin=[]  FilterOutMax=[]  SumOutMin=[]  SumOutMax=[]  SumI1OutMin=[]  SumI1OutMax=[]  SumI2OutMin=[]  SumI2OutMax=[]  SumI3OutMin=[]  SumI3OutMax=[]  SumDOutMin=[]  SumDOutMax=[]  SaturationOutMin=[]  SaturationOutMax=[]  IntegratorContinuousStateAttributes=''  IntegratorStateMustResolveToSignalObject=off  IntegratorRTWStateStorageClass=Auto  FilterContinuousStateAttributes=''  FilterStateMustResolveToSignalObject=off  FilterRTWStateStorageClass=Auto  DifferentiatorICPrevScaledInput=0  DifferentiatorOutMin=[]  DifferentiatorOutMax=[]
  PID Controller4 : simulink/Continuous/PID Controller  Controller=PD  TimeDomain=Discrete-time  SampleTime=Tc  IntegratorMethod=Forward Euler  FilterMethod=Forward Euler  Form=Parallel  UseFilter=off  ControllerParametersSource=internal  P=2.6  I=2.36803176515497  D=0  N=3.83298618768959  InitialConditionSource=internal  InitialConditionForIntegrator=0  InitialConditionForFilter=0  ExternalReset=none  LimitOutput=off  UpperSaturationLimit=inf  LowerSaturationLimit=-inf  LinearizeAsGain=on  AntiWindupMode=none  Kb=1  TrackingMode=off  Kt=1  PParamMin=[]  PParamMax=[]  IParamMin=[]  IParamMax=[]  DParamMin=[]  DParamMax=[]  NParamMin=[]  NParamMax=[]  KbParamMin=[]  KbParamMax=[]  KtParamMin=[]  KtParamMax=[]  POutMin=[]  POutMax=[]  IOutMin=[]  IOutMax=[]  DOutMin=[]  DOutMax=[]  NOutMin=[]  NOutMax=[]  KbOutMin=[]  KbOutMax=[]  KtOutMin=[]  KtOutMax=[]  IntegratorOutMin=[]  IntegratorOutMax=[]  FilterOutMin=[]  FilterOutMax=[]  SumOutMin=[]  SumOutMax=[]  SumI1OutMin=[]  SumI1OutMax=[]  SumI2OutMin=[]  SumI2OutMax=[]  SumI3OutMin=[]  SumI3OutMax=[]  SumDOutMin=[]  SumDOutMax=[]  SaturationOutMin=[]  SaturationOutMax=[]  IntegratorContinuousStateAttributes=''  IntegratorStateMustResolveToSignalObject=off  IntegratorRTWStateStorageClass=Auto  FilterContinuousStateAttributes=''  FilterStateMustResolveToSignalObject=off  FilterRTWStateStorageClass=Auto  DifferentiatorICPrevScaledInput=0  DifferentiatorOutMin=[]  DifferentiatorOutMax=[]
  PID Controller5 : simulink/Continuous/PID Controller  Controller=PD  TimeDomain=Discrete-time  SampleTime=Tq  IntegratorMethod=Forward Euler  FilterMethod=Forward Euler  Form=Parallel  UseFilter=off  ControllerParametersSource=internal  P=15  I=35.1207902652377  D=0.2  N=40.0107970227961  InitialConditionSource=internal  InitialConditionForIntegrator=0  InitialConditionForFilter=0  ExternalReset=none  LimitOutput=off  UpperSaturationLimit=inf  LowerSaturationLimit=-inf  LinearizeAsGain=on  AntiWindupMode=none  Kb=1  TrackingMode=off  Kt=1  PParamMin=[]  PParamMax=[]  IParamMin=[]  IParamMax=[]  DParamMin=[]  DParamMax=[]  NParamMin=[]  NParamMax=[]  KbParamMin=[]  KbParamMax=[]  KtParamMin=[]  KtParamMax=[]  POutMin=[]  POutMax=[]  IOutMin=[]  IOutMax=[]  DOutMin=[]  DOutMax=[]  NOutMin=[]  NOutMax=[]  KbOutMin=[]  KbOutMax=[]  KtOutMin=[]  KtOutMax=[]  IntegratorOutMin=[]  IntegratorOutMax=[]  FilterOutMin=[]  FilterOutMax=[]  SumOutMin=[]  SumOutMax=[]  SumI1OutMin=[]  SumI1OutMax=[]  SumI2OutMin=[]  SumI2OutMax=[]  SumI3OutMin=[]  SumI3OutMax=[]  SumDOutMin=[]  SumDOutMax=[]  SaturationOutMin=[]  SaturationOutMax=[]  IntegratorContinuousStateAttributes=''  IntegratorStateMustResolveToSignalObject=off  IntegratorRTWStateStorageClass=Auto  FilterContinuousStateAttributes=''  FilterStateMustResolveToSignalObject=off  FilterRTWStateStorageClass=Auto  DifferentiatorICPrevScaledInput=0  DifferentiatorOutMin=[]  DifferentiatorOutMax=[]
  PID Controller7 : simulink/Continuous/PID Controller  Controller=PID  TimeDomain=Discrete-time  SampleTime=Tc  IntegratorMethod=Forward Euler  FilterMethod=Forward Euler  Form=Parallel  UseFilter=on  ControllerParametersSource=internal  P=0.015  I=0  D=0.25  N=3  InitialConditionSource=internal  InitialConditionForIntegrator=0  InitialConditionForFilter=0  ExternalReset=none  LimitOutput=off  UpperSaturationLimit=inf  LowerSaturationLimit=-inf  LinearizeAsGain=on  AntiWindupMode=none  Kb=1  TrackingMode=off  Kt=1  PParamMin=[]  PParamMax=[]  IParamMin=[]  IParamMax=[]  DParamMin=[]  DParamMax=[]  NParamMin=[]  NParamMax=[]  KbParamMin=[]  KbParamMax=[]  KtParamMin=[]  KtParamMax=[]  POutMin=[]  POutMax=[]  IOutMin=[]  IOutMax=[]  DOutMin=[]  DOutMax=[]  NOutMin=[]  NOutMax=[]  KbOutMin=[]  KbOutMax=[]  KtOutMin=[]  KtOutMax=[]  IntegratorOutMin=[]  IntegratorOutMax=[]  FilterOutMin=[]  FilterOutMax=[]  SumOutMin=[]  SumOutMax=[]  SumI1OutMin=[]  SumI1OutMax=[]  SumI2OutMin=[]  SumI2OutMax=[]  SumI3OutMin=[]  SumI3OutMax=[]  SumDOutMin=[]  SumDOutMax=[]  SaturationOutMin=[]  SaturationOutMax=[]  IntegratorContinuousStateAttributes=''  IntegratorStateMustResolveToSignalObject=off  IntegratorRTWStateStorageClass=Auto  FilterContinuousStateAttributes=''  FilterStateMustResolveToSignalObject=off  FilterRTWStateStorageClass=Auto  DifferentiatorICPrevScaledInput=0  DifferentiatorOutMin=[]  DifferentiatorOutMax=[]
  PID Controller9 : simulink/Continuous/PID Controller  Controller=PD  TimeDomain=Discrete-time  SampleTime=Tq  IntegratorMethod=Forward Euler  FilterMethod=Forward Euler  Form=Parallel  UseFilter=off  ControllerParametersSource=internal  P=4600  I=1575.82088970639  D=550  N=244.660686071579  InitialConditionSource=internal  InitialConditionForIntegrator=0  InitialConditionForFilter=0  ExternalReset=none  LimitOutput=off  UpperSaturationLimit=inf  LowerSaturationLimit=-inf  LinearizeAsGain=on  AntiWindupMode=none  Kb=1  TrackingMode=off  Kt=1  PParamMin=[]  PParamMax=[]  IParamMin=[]  IParamMax=[]  DParamMin=[]  DParamMax=[]  NParamMin=[]  NParamMax=[]  KbParamMin=[]  KbParamMax=[]  KtParamMin=[]  KtParamMax=[]  POutMin=[]  POutMax=[]  IOutMin=[]  IOutMax=[]  DOutMin=[]  DOutMax=[]  NOutMin=[]  NOutMax=[]  KbOutMin=[]  KbOutMax=[]  KtOutMin=[]  KtOutMax=[]  IntegratorOutMin=[]  IntegratorOutMax=[]  FilterOutMin=[]  FilterOutMax=[]  SumOutMin=[]  SumOutMax=[]  SumI1OutMin=[]  SumI1OutMax=[]  SumI2OutMin=[]  SumI2OutMax=[]  SumI3OutMin=[]  SumI3OutMax=[]  SumDOutMin=[]  SumDOutMax=[]  SaturationOutMin=[]  SaturationOutMax=[]  IntegratorContinuousStateAttributes=''  IntegratorStateMustResolveToSignalObject=off  IntegratorRTWStateStorageClass=Auto  FilterContinuousStateAttributes=''  FilterStateMustResolveToSignalObject=off  FilterRTWStateStorageClass=Auto  DifferentiatorICPrevScaledInput=0  DifferentiatorOutMin=[]  DifferentiatorOutMax=[]
  Pitch Controller Input : Subsystem  Variant=on
  Pitch Rate Controller Input : Subsystem  Variant=on
  Roll Controller Input : Subsystem  Variant=on
  Roll Rate Controller Input : Subsystem  Variant=on
  Saturation{,1..3} (4 alike) : Saturate  UpperLimit=20000  LowerLimit=-20000
  Scope{1..4,6,9,11..13} (9 alike) : Scope
  Sum{1..5,7,9..11} (9 alike) : Sum  Inputs=|+-
  To Workspace : ToWorkspace  VariableName=pitch_setpoint_model  SaveFormat=Structure With Time  SampleTime=-1
  To Workspace1 : ToWorkspace  VariableName=pitchrate_setpoint_model  SaveFormat=Structure With Time  SampleTime=Tq
  To Workspace10 : ToWorkspace  VariableName=yaw_value_model  SaveFormat=Structure With Time  SampleTime=Tc
  To Workspace11 : ToWorkspace  VariableName=y_position_model  SaveFormat=Structure With Time  SampleTime=Tc
  To Workspace12 : ToWorkspace  VariableName=z_position_model  SaveFormat=Structure With Time  SampleTime=Tc
  To Workspace2 : ToWorkspace  VariableName=x_command_model  SaveFormat=Structure With Time  SampleTime=Tq
  To Workspace3 : ToWorkspace  VariableName=roll_setpoint_model  SaveFormat=Structure With Time  SampleTime=Tc
  To Workspace4 : ToWorkspace  VariableName=rollrate_setpoint_model  SaveFormat=Structure With Time  SampleTime=Tq
  To Workspace5 : ToWorkspace  VariableName=y_command_model  SaveFormat=Structure With Time  SampleTime=Tq
  To Workspace6 : ToWorkspace  VariableName=z_command_model  SaveFormat=Structure With Time  SampleTime=Tq
  To Workspace7 : ToWorkspace  VariableName=yawrate_setpoint_model  SaveFormat=Structure With Time  SampleTime=Tc
  To Workspace8 : ToWorkspace  VariableName=yaw_command_model  SaveFormat=Structure With Time  SampleTime=Tq
  To Workspace9 : ToWorkspace  VariableName=x_position_model  SaveFormat=Structure With Time  SampleTime=Tc
  Yaw Controller Input : Subsystem  Variant=on
  Yaw Rate Controller Input : Subsystem  Variant=on
  height_controlled : Outport
  y_controlled : Outport  Port=2
  x_controlled : Outport  Port=3
  yaw_controlled : Outport  Port=4
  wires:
  pitch_rate/1 -> Scope6/1, Sum4/2
  z_setpoint/1 -> Sum7/1
  x_position/1 -> Scope4/1, To Workspace9/1, Sum5/2
  PID Controller5/1 -> Sum4/1, To Workspace1/1
  PID Controller11/1 -> Sum3/1, To Workspace/1
  pitch/1 -> Gain/1, Sum3/2
  Gain/1 -> Scope9/1
  PID Controller1/1 -> To Workspace8/1, Saturation/1
  PID Controller9/1 -> To Workspace2/1, Saturation1/1
  Latitude Controller Input/1(x_error) -> PID Controller11/1
  x_setpoint/1 -> Sum5/1
  roll_rate/1 -> Scope11/1, Sum10/2
  y_position/1 -> Scope12/1, To Workspace11/1, Sum11/2
  PID Controller2/1 -> Sum10/1, To Workspace4/1
  PID Controller7/1 -> Sum9/1, To Workspace3/1
  roll/1 -> Gain2/1, Sum9/2
  Gain2/1 -> Scope13/1
  y_setpoint/1 -> Sum11/1
  PID Controller17/1 -> To Workspace6/1, Saturation3/1
  yaw/1 -> Scope3/1, To Workspace10/1, Sum1/2
  yaw_setpoint/1 -> Sum1/1
  yaw_rate/1 -> Gain1/1, Sum2/2
  Gain1/1 -> Scope1/1
  PID Controller4/1 -> Sum2/1, To Workspace7/1
  z_position/1 -> To Workspace12/1, Scope2/1, Sum7/2
  Sum1/1 -> Yaw Controller Input/1(yaw_error_model)
  Yaw Controller Input/1(yaw_error) -> PID Controller4/1
  Sum2/1 -> Yaw Rate Controller Input/1(yawrate_error_model)
  Yaw Rate Controller Input/1(yawrate_error) -> PID Controller1/1
  Sum5/1 -> Latitude Controller Input/1(x_error_model)
  Sum3/1 -> Pitch Controller Input/1(pitch_error_model)
  Pitch Controller Input/1(pitch_error) -> PID Controller5/1
  Sum4/1 -> Pitch Rate Controller Input/1(pitchrate_error_model)
  Pitch Rate Controller Input/1(pitchrate_error) -> PID Controller9/1
  Sum11/1 -> Longitude Controller Input/1(y_error_model)
  Longitude Controller Input/1(y_error) -> PID Controller7/1
  Sum9/1 -> Roll Controller Input/1(roll_error_model)
  Roll Controller Input/1(roll_error) -> PID Controller2/1
  Sum10/1 -> Roll Rate Controller Input/1(rollrate_error_model)
  Altitude Controller Input/1(z_error) -> PID Controller17/1
  Sum7/1 -> Altitude Controller Input/1(z_error_model)
  Roll Rate Controller Input/1(rollrate_error) -> PID Controller3/1
  PID Controller3/1 -> To Workspace5/1, Saturation2/1
  Saturation2/1 -> y_controlled/1
  Saturation1/1 -> x_controlled/1
  Saturation/1 -> yaw_controlled/1

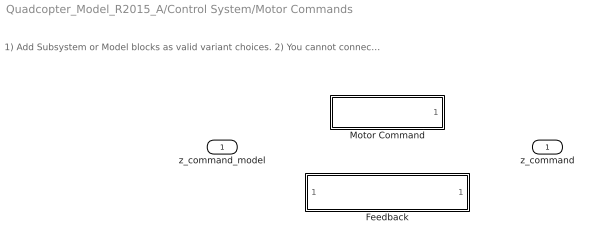
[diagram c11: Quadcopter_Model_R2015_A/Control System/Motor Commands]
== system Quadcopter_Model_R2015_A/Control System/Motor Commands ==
  note: 1) Add Subsystem or Model blocks as valid variant choices. 2) You cannot connect blocks at this level. At simulation, connectivity is automatically determined, based on the active variant and port name matching.
  z_command_model : Inport
  Feedback : Subsystem  VariantControl=logAnalysisToggle==0
  Motor Command : Subsystem  VariantControl=logAnalysisToggle==1
  z_command : Outport

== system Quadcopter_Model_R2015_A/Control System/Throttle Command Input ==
  note: 1) Add Subsystem or Model blocks as valid variant choices. 2) You cannot connect blocks at this level. At simulation, connectivity is automatically determined, based on the active variant and port name matching.
  z_command_model : Inport
  Feedback : Subsystem  VariantControl=logAnalysisToggle==0
  Throttle Command : Subsystem  VariantControl=logAnalysisToggle==1
  z_command : Outport

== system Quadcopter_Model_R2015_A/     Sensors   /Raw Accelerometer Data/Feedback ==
  raw_accel_model : Inport
  raw_accel : Outport
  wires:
  raw_accel_model/1 -> raw_accel/1

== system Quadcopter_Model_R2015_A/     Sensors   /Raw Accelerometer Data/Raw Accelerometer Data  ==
  From Workspace5 : FromWorkspace  VariableName=raw_accel_data  SampleTime=Tq
  raw_accel : Outport
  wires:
  From Workspace5/1 -> raw_accel/1

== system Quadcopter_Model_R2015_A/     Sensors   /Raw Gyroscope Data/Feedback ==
  raw_gyro_model : Inport
  raw_gyro : Outport
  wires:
  raw_gyro_model/1 -> raw_gyro/1

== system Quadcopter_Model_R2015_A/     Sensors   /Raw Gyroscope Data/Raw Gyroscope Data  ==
  From Workspace5 : FromWorkspace  VariableName=raw_accel_data  SampleTime=Tq
  raw_gyro : Outport
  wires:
  From Workspace5/1 -> raw_gyro/1

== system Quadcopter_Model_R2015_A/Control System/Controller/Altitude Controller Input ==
  note: 1) Add Subsystem or Model blocks as valid variant choices. 2) You cannot connect blocks at this level. At simulation, connectivity is automatically determined, based on the active variant and port name matching.
  z_error_model : Inport
  Feedback : Subsystem  VariantControl=logAnalysisToggle==0
  z error : Subsystem  VariantControl=logAnalysisToggle==1
  z_error : Outport

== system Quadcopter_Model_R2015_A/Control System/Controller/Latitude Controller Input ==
  note: 1) Add Subsystem or Model blocks as valid variant choices. 2) You cannot connect blocks at this level. At simulation, connectivity is automatically determined, based on the active variant and port name matching.
  x_error_model : Inport
  Feedback : Subsystem  VariantControl=logAnalysisToggle==0
  x error : Subsystem  VariantControl=logAnalysisToggle==1
  x_error : Outport

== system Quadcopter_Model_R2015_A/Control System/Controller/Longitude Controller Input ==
  note: 1) Add Subsystem or Model blocks as valid variant choices. 2) You cannot connect blocks at this level. At simulation, connectivity is automatically determined, based on the active variant and port name matching.
  y_error_model : Inport
  Feedback : Subsystem  VariantControl=logAnalysisToggle==0
  y error : Subsystem  VariantControl=logAnalysisToggle==1
  y_error : Outport

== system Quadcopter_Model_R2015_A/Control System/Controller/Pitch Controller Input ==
  note: 1) Add Subsystem or Model blocks as valid variant choices. 2) You cannot connect blocks at this level. At simulation, connectivity is automatically determined, based on the active variant and port name matching.
  pitch_error_model : Inport
  Feedback : Subsystem  VariantControl=logAnalysisToggle==0
  pitch error : Subsystem  VariantControl=logAnalysisToggle==1
  pitch_error : Outport

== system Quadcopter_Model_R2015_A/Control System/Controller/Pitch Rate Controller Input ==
  note: 1) Add Subsystem or Model blocks as valid variant choices. 2) You cannot connect blocks at this level. At simulation, connectivity is automatically determined, based on the active variant and port name matching.
  pitchrate_error_model : Inport
  Feedback : Subsystem  VariantControl=logAnalysisToggle==0
  pitchrate error : Subsystem  VariantControl=logAnalysisToggle==1
  pitchrate_error : Outport

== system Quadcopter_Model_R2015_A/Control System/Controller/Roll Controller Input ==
  note: 1) Add Subsystem or Model blocks as valid variant choices. 2) You cannot connect blocks at this level. At simulation, connectivity is automatically determined, based on the active variant and port name matching.
  roll_error_model : Inport
  Feedback : Subsystem  VariantControl=logAnalysisToggle==0
  roll error : Subsystem  VariantControl=logAnalysisToggle==1
  roll_error : Outport

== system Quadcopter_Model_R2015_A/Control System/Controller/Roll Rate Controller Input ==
  note: 1) Add Subsystem or Model blocks as valid variant choices. 2) You cannot connect blocks at this level. At simulation, connectivity is automatically determined, based on the active variant and port name matching.
  rollrate_error_model : Inport
  Feedback : Subsystem  VariantControl=logAnalysisToggle==0
  rollrate error : Subsystem  VariantControl=logAnalysisToggle==1
  rollrate_error : Outport

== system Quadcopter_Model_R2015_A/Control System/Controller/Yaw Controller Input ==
  note: 1) Add Subsystem or Model blocks as valid variant choices. 2) You cannot connect blocks at this level. At simulation, connectivity is automatically determined, based on the active variant and port name matching.
  yaw_error_model : Inport
  Feedback : Subsystem  VariantControl=logAnalysisToggle==0
  yaw error : Subsystem  VariantControl=logAnalysisToggle==1
  yaw_error : Outport

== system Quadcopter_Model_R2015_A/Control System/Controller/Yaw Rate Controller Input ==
  note: 1) Add Subsystem or Model blocks as valid variant choices. 2) You cannot connect blocks at this level. At simulation, connectivity is automatically determined, based on the active variant and port name matching.
  yawrate_error_model : Inport
  Feedback : Subsystem  VariantControl=logAnalysisToggle==0
  yawrate error : Subsystem  VariantControl=logAnalysisToggle==1
  yawrate_error : Outport

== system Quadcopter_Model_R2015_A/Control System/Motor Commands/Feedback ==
  z_command_model : Inport
  z_command : Outport
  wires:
  z_command_model/1 -> z_command/1

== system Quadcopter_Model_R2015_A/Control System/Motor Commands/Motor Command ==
  From Workspace5 : FromWorkspace  VariableName=motor_commands  SampleTime=Tq
  z_command : Outport
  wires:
  From Workspace5/1 -> z_command/1

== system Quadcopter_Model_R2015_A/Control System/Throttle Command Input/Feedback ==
  z_command_model : Inport
  z_command : Outport
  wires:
  z_command_model/1 -> z_command/1

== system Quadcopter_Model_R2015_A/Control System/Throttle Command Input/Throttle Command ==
  From Workspace5 : FromWorkspace  VariableName=throttle_command  SampleTime=Tq
  z_command : Outport
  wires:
  From Workspace5/1 -> z_command/1

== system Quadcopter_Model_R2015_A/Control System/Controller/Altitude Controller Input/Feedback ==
  z_error_model : Inport
  z_error : Outport
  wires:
  z_error_model/1 -> z_error/1

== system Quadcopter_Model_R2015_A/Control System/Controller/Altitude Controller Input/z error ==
  From Workspace6 : FromWorkspace  VariableName=z_error  SampleTime=Tc
  z_error : Outport
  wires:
  From Workspace6/1 -> z_error/1

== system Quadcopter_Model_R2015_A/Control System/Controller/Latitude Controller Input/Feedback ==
  x_error_model : Inport
  x_error : Outport
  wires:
  x_error_model/1 -> x_error/1

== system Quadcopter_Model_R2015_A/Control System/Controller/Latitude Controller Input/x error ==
  From Workspace : FromWorkspace  VariableName=x_error  SampleTime=Tc
  x_error : Outport
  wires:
  From Workspace/1 -> x_error/1

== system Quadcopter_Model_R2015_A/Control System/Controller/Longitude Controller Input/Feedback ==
  y_error_model : Inport
  y_error : Outport
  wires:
  y_error_model/1 -> y_error/1

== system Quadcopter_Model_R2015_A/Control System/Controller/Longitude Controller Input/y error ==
  From Workspace3 : FromWorkspace  VariableName=y_error  SampleTime=Tc
  y_error : Outport
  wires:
  From Workspace3/1 -> y_error/1

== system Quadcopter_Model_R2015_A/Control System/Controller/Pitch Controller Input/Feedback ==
  pitch_error_model : Inport
  pitch_error : Outport
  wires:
  pitch_error_model/1 -> pitch_error/1

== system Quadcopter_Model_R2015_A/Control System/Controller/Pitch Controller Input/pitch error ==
  From Workspace : FromWorkspace  VariableName=pitch_error  SampleTime=Tq
  pitch_error : Outport
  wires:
  From Workspace/1 -> pitch_error/1

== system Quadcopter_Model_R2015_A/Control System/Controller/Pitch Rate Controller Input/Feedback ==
  pitchrate_error_model : Inport
  pitchrate_error : Outport
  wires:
  pitchrate_error_model/1 -> pitchrate_error/1
